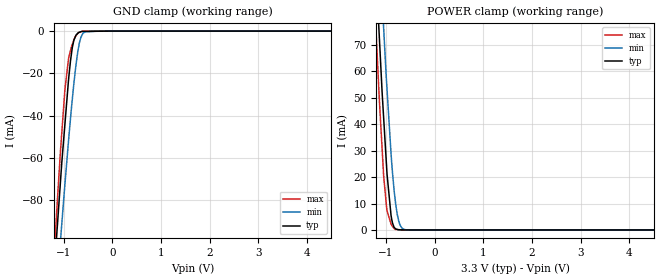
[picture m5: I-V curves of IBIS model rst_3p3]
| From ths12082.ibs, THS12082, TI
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|   rst_3p3 Model
[Model]   rst_3p3
Model_type   Input
Vinl = 0.6
Vinh = 2
|   typ   min   max
|   (nom PVT)   (fast PVT)   (slow PVT)
C_comp   1.065e-12   1.052e-12   1.069e-12
| Where nom  PVT is Nominal Process, 3.3V, 27C
|   Fast PVT is Strong Process,  3.6V, -55C
|   Slow PVT is Weak Process,   3V, 125C
[Voltage Range]   3.3   3   3.6
|Ambient Temperature   25   125   -55
|Junction Temperature
[Temperature Range]   27   125   -55
[Power Clamp Reference]   3.3   3   3.6
[GND Clamp Reference]   0   0   0
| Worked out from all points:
|   GND clamp passes 1 mA (typ) near -0.71 V on its own axis
|   POWER clamp passes 1 mA (typ) near -0.83 V on its own axis
[GND Clamp]
|   Voltage   I(typ)   I(min)   I(max)
-3.3V     -936.4mA   -898.3mA   -1.01A
-1.224V   -123.9mA   -149mA     -116.9mA
-1.084V   -77.76mA   -105.2mA   -63.93mA
-1.036V   -62.21mA   -91.13mA   -48.07mA
-972mV    -44.03mA   -72.36mA   -27.61mA
-896.4mV  -22.71mA   -51.46mA   -12.83mA
-858mV    -14.19mA   -41.45mA   -9.321mA
-792mV    -4.698mA   -25.64mA   -4.371mA
-696.3mV  -755.2uA   -8.26mA    -766.1uA
-591mV    -157.9uA   -849.9uA   -44.18uA
-285mV    -75.68uA   -318.2nA   -33.34nA
6.6V      0A         0A         0A
[POWER Clamp]
|   Voltage   I(typ)   I(min)   I(max)
-3.3V     964mA      977.7mA    963.7mA
-1.247V   112.8mA    148.4mA    91.47mA
-1.145V   75.37mA    109.6mA    51.9mA
-1.082V   52.61mA    87.7mA     31.18mA
-1.048V   41.84mA    75.7mA     20.05mA
-982.8mV  21.99mA    54.01mA    7.396mA
-897.6mV  5.51mA     28.89mA    2.236mA
-813.6mV  603.3uA    11.58mA    241.2uA
-768mV    202.8uA    5.73mA     132.6uA
-711mV    51.94uA    1.788mA    84.44uA
-591mV    9.743uA    71.91uA    14.59uA
6.6V      0A         0A         0A
